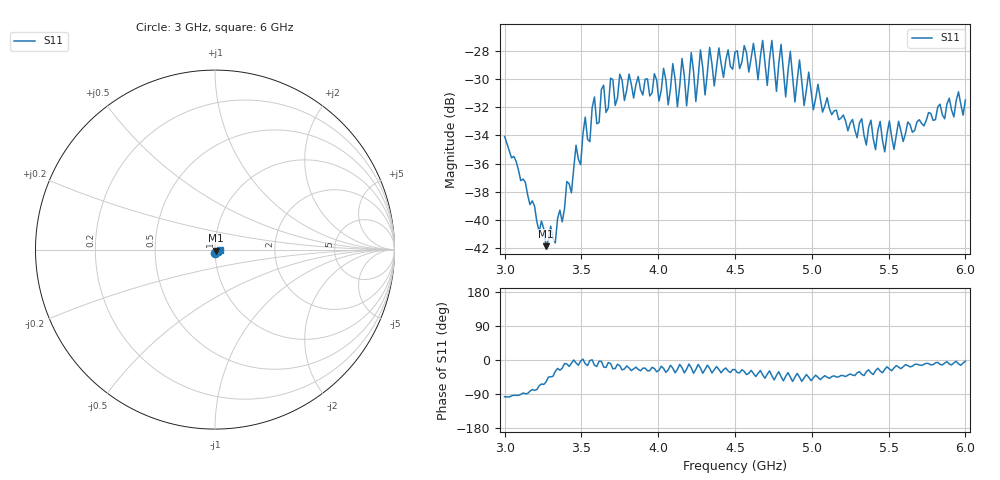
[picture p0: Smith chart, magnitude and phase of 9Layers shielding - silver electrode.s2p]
!  03/07/2025  17:12:23
! Ref Plane: 0.000 mm
# MHZ S MA R  50
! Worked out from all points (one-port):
!   201 points, 3 GHz to 6 GHz, reference 50 ohm
!   lowest |S11| = -41.8 dB at 3.27 GHz (marker M1), VSWR 1.02, Z = 50.4 - j0.691 ohm
!   |S11| at or under -10 dB: start of sweep to end of sweep
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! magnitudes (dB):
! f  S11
! 3 GHz  -34.1
! 3.27 GHz  -41.8
! 3.375 GHz  -40.1
! 3.525 GHz  -32.7
! 3.555 GHz  -34.4
! 3.585 GHz  -31.3
! 3.615 GHz  -33.1
! 3.75 GHz  -29.7
! 4.005 GHz  -31.6
! 4.035 GHz  -29.3
! 4.065 GHz  -31.8
! 4.095 GHz  -28.9
! 4.125 GHz  -32.0
! 4.155 GHz  -28.6
! 4.185 GHz  -31.9
! 4.215 GHz  -28.1
! 4.245 GHz  -31.6
! 4.275 GHz  -28.0
! 4.305 GHz  -31.1
! 4.335 GHz  -27.8
! 4.365 GHz  -30.5
! 4.395 GHz  -27.8
! 4.5 GHz  -28.1
! 4.875 GHz  -29.8
! 5.25 GHz  -33.1
! 5.475 GHz  -35.2
! 5.625 GHz  -33.1
! 6 GHz  -31.5
